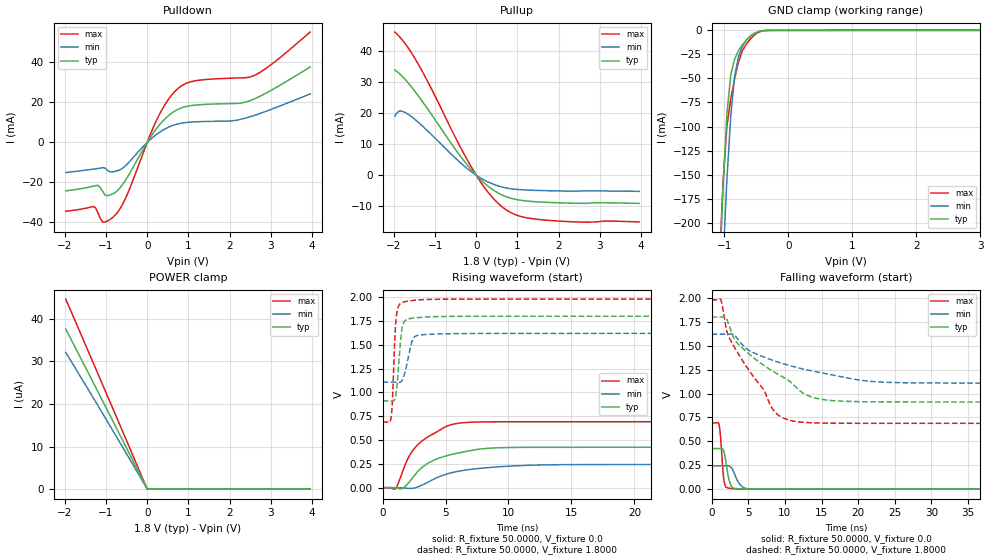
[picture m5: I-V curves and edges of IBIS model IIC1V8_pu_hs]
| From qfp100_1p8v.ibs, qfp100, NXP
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[Model] IIC1V8_pu_hs
|   Model IIC1V8_pu_hs
| This model was characterised for following simulation conditions:
| External (pad) voltage:
|   - Typ: 1.8V,   - Min: 1.62V,   - Max: 1.98V
| Library cells for typ/min/max conditions are connected as defined below:
|  IO - External Pad
|  A - Core Input
|  EN - Output Buffer Enable
|  BOOST - vdde
|  EGP - vdd
|  EHS - vdd
|  ENZI - vdd
|  EPD - gnd
|  EPUN - gnd
|  ZI - NC
|  ZIF - NC
|  gnd - gnd
|  gnde - gnde
|  vdd - vdd
|  vdde - vdde
| All other pins connected to ground
Model_type I/O
Polarity   Non-Inverting
Enable   Active-Low
Vinl =   0.5400V
Vinh =   1.2600V
Vmeas =  0.9000V
Cref =   0.0F
Rref =   1.0000k
Vref =   0.0V
C_comp   3.6100pF   3.4623pF   3.7513pF
|C_comp_pullup   0.9281pF   0.9064pF   0.9342pF
|C_comp_pulldown   2.3311pF   2.4845pF   2.1852pF
[Model Spec]
| variable   typ   min   max
Vinh   0.5400V   0.4860V   0.5940V
Vinl   1.2600V   1.1340V   1.3860V
Vmeas   0.9000V   0.8100V   0.9900V
[Temperature Range]   25.0000   0.1250k   -40.0000
[Voltage Range]   1.8000V   1.6200V   1.9800V
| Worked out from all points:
|   slope of the pulldown table from 0 to 0.27 V, typ, clamps not added: 33.4 ohm
|   slope of the pullup table from 0 to 0.27 V, typ, clamps not added: 80.7 ohm
|   GND clamp passes 1 mA (typ) near -0.44 V on its own axis
|   rising waveform, R_fixture 50.0000, V_fixture 0.0: 20-80 % time 2.94ns typ, 3.7ns min, 2.37ns max; typ from 0.001 V to 0.424 V
|   rising waveform, R_fixture 50.0000, V_fixture 1.8000: 20-80 % time 334ps typ, 514ps min, 244ps max; typ from 0.912 V to 1.8 V
|   falling waveform, R_fixture 50.0000, V_fixture 0.0: 20-80 % time 583ps typ, 940ps min, 400ps max; typ from 0.424 V to 0.001 V
|   falling waveform, R_fixture 50.0000, V_fixture 1.8000: 20-80 % time 8.42ns typ, 11.2ns min, 5.75ns max; typ from 1.8 V to 0.912 V
[Pulldown]
|Voltage   I(typ)   I(min)   I(max)
-1.98V    -24.22mA   -15.04mA   -34.42mA
-1.32V    -21.94mA   -13.41mA   -32.06mA
-1.2V     -21.45mA   -13.05mA   -35.06mA
-1.08V    -24.63mA   -12.6mA    -39.9mA
-900mV    -26.23mA   -14.78mA   -38.53mA
-720mV    -24.07mA   -14.13mA   -34.99mA
-540mV    -19.33mA   -11.9mA    -28.53mA
300mV     8.856mA    5.096mA    14.12mA
720mV     16.26mA    9.117mA    26.48mA
1.14V     18.6mA     10.26mA    30.69mA
2.58V     21.55mA    13.34mA    33.32mA
3.96V     37.7mA     24.26mA    55.17mA
[Pullup]
|Voltage   I(typ)   I(min)   I(max)
-1.98V    33.82mA    18.95mA    45.98mA
-1.86V    32.54mA    20.66mA    44.41mA
-1.62V    29.1mA     19.25mA    40.23mA
-1.2V     21.63mA    14.45mA    30.58mA
-420mV    6.731mA    4.413mA    9.887mA
0V        252.9fA    74.02pA    -178.3fA
360mV     -4.265mA   -2.608mA   -6.666mA
660mV     -6.57mA    -3.917mA   -10.5mA
1.02V     -7.945mA   -4.606mA   -13.01mA
1.56V     -8.618mA   -4.934mA   -14.29mA
2.64V     -9.058mA   -5.064mA   -15.11mA
3.96V     -9.081mA   -5.209mA   -15.04mA
[GND_clamp]
|Voltage   I(typ)   I(min)   I(max)
-1.98V    -2.104A    -2.075A    -2.136A
-1.08V    -259.3mA   -333mA     -247mA
-1.02V    -161.8mA   -238.7mA   -157.2mA
-960mV    -86.78mA   -154.8mA   -99.51mA
-900mV    -45.99mA   -88.85mA   -71.1mA
-840mV    -29.94mA   -48.03mA   -50.31mA
-780mV    -21.2mA    -27.67mA   -33.04mA
-720mV    -15.2mA    -16.91mA   -21.32mA
-660mV    -10.61mA   -10.27mA   -14.61mA
-540mV    -3.83mA    -3.432mA   -5.346mA
-300mV    -56.31uA   -67.68uA   -68.13uA
3.96V     0A         0A         0A
[POWER_clamp]
|Voltage   I(typ)   I(min)   I(max)
-1.98V    37.59uA    32.11uA    44.63uA
-960mV    18.36uA    15.76uA    21.73uA
0V        104.7pA    4.893nA    11.38pA
3.96V     0A         0A         0A
[Ramp]
| variable   typ   min   max
dV/dt_r  0.2543/2.9378n   0.1460/3.6987n   0.4154/2.3696n
dV/dt_f  0.5330/8.4184n   0.3064/11.2418n   0.7749/5.7473n
R_load = 50.0000
[Rising Waveform]
R_fixture= 50.0000
V_fixture= 0.0
V_fixture_min= 0.0
V_fixture_max= 0.0
|time   V(typ)   V(min)   V(max)
0s        634.5uV    668.6uV    603.2uV
1.053ns   -3.814mV   909.4uV    -8.132mV
1.609ns   -7.22mV    -1.607mV   175.8mV
2.272ns   85.08mV    -8.002mV   366.5mV
2.949ns   191.3mV    16.1mV     469.6mV
3.634ns   259.1mV    60.26mV    535.9mV
5.668ns   354.5mV    162.9mV    668mV
8.815ns   417.3mV    215.8mV    691.9mV
23.03ns   424.4mV    243.8mV    692.9mV
1us       424.5mV    243.9mV    693mV
[Rising Waveform]
R_fixture= 50.0000
V_fixture= 1.8000
V_fixture_min= 1.6200
V_fixture_max= 1.9800
|time   V(typ)   V(min)   V(max)
0s        911.7mV    1.109V     688.6mV
690.5ps   909.6mV    1.11V      744.3mV
788.8ps   906.6mV    1.11V      924.6mV
1.019ns   952.3mV    1.108V     1.681V
1.284ns   1.297V     1.103V     1.91V
1.514ns   1.644V     1.12V      1.942V
1.777ns   1.752V     1.209V     1.953V
2.535ns   1.782V     1.584V     1.968V
4.889ns   1.798V     1.615V     1.979V
1us       1.8V       1.62V      1.98V
[Falling Waveform]
R_fixture= 50.0000
V_fixture= 0.0
V_fixture_min= 0.0
V_fixture_max= 0.0
|time   V(typ)   V(min)   V(max)
0s        424.5mV    243.9mV    693mV
1.025ns   424.6mV    243.9mV    675mV
1.232ns   427.2mV    243.9mV    538.3mV
1.606ns   408.7mV    244mV      144.6mV
1.875ns   327mV      245.4mV    33.23mV
2.341ns   111.1mV    244.7mV    11.87mV
2.757ns   25.93mV    219.5mV    6.599mV
3.715ns   4.605mV    65.74mV    2.39mV
4.705ns   2.126mV    7.934mV    1.234mV
1us       634.5uV    668.7uV    603.2uV
[Falling Waveform]
R_fixture= 50.0000
V_fixture= 1.8000
V_fixture_min= 1.6200
V_fixture_max= 1.9800
|time   V(typ)   V(min)   V(max)
0s        1.8V       1.62V      1.98V
1.241ns   1.8V       1.62V      1.984V
1.932ns   1.799V     1.62V      1.702V
2.447ns   1.699V     1.622V     1.578V
3.741ns   1.51V      1.552V     1.404V
8.587ns   1.223V     1.341V     812.8mV
12.83ns   990.2mV    1.251V     697.8mV
15.55ns   934mV      1.209V     690.8mV
35ns      912.1mV    1.11V      688.7mV
1us       911.7mV    1.109V     688.6mV
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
